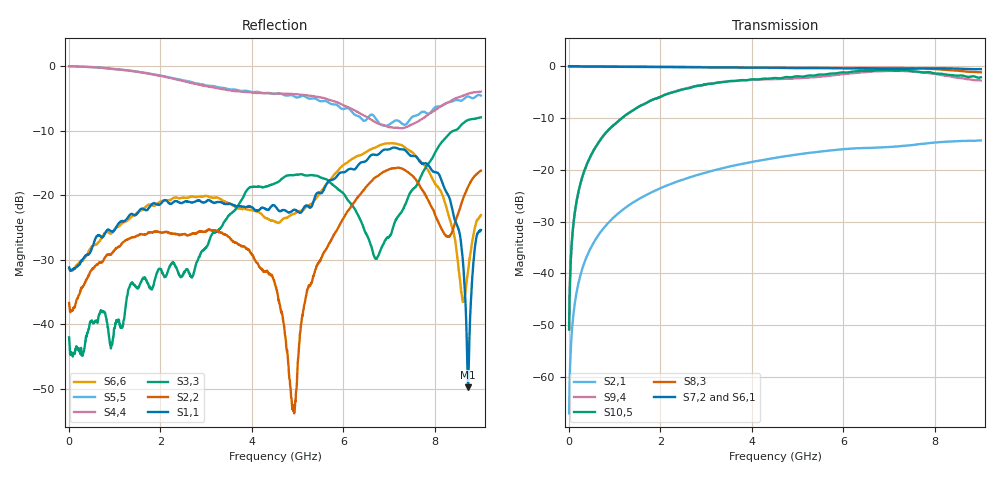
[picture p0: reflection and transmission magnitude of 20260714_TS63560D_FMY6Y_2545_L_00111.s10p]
# GHz S DB R 50
! CMT, SN0916, 25263762, 26.7.0
! Date: 15.07.2026 13:36:52
! Data: Format
! Freq S1.1:dB/Ang S1.2:dB/Ang S1.3:dB/Ang S1.4:dB/Ang S1.5:dB/Ang S1.6:dB/Ang S1.7:dB/Ang S1.8:dB/Ang S1.9:dB/Ang S1.10:dB/Ang
!  S2.1:dB/Ang S2.2:dB/Ang S2.3:dB/Ang S2.4:dB/Ang S2.5:dB/Ang S2.6:dB/Ang S2.7:dB/Ang S2.8:dB/Ang S2.9:dB/Ang S2.10:dB/Ang
!  S3.1:dB/Ang S3.2:dB/Ang S3.3:dB/Ang S3.4:dB/Ang S3.5:dB/Ang S3.6:dB/Ang S3.7:dB/Ang S3.8:dB/Ang S3.9:dB/Ang S3.10:dB/Ang
!  S4.1:dB/Ang S4.2:dB/Ang S4.3:dB/Ang S4.4:dB/Ang S4.5:dB/Ang S4.6:dB/Ang S4.7:dB/Ang S4.8:dB/Ang S4.9:dB/Ang S4.10:dB/Ang
!  S5.1:dB/Ang S5.2:dB/Ang S5.3:dB/Ang S5.4:dB/Ang S5.5:dB/Ang S5.6:dB/Ang S5.7:dB/Ang S5.8:dB/Ang S5.9:dB/Ang S5.10:dB/Ang
!  S6.1:dB/Ang S6.2:dB/Ang S6.3:dB/Ang S6.4:dB/Ang S6.5:dB/Ang S6.6:dB/Ang S6.7:dB/Ang S6.8:dB/Ang S6.9:dB/Ang S6.10:dB/Ang
!  S7.1:dB/Ang S7.2:dB/Ang S7.3:dB/Ang S7.4:dB/Ang S7.5:dB/Ang S7.6:dB/Ang S7.7:dB/Ang S7.8:dB/Ang S7.9:dB/Ang S7.10:dB/Ang
!  S8.1:dB/Ang S8.2:dB/Ang S8.3:dB/Ang S8.4:dB/Ang S8.5:dB/Ang S8.6:dB/Ang S8.7:dB/Ang S8.8:dB/Ang S8.9:dB/Ang S8.10:dB/Ang
!  S9.1:dB/Ang S9.2:dB/Ang S9.3:dB/Ang S9.4:dB/Ang S9.5:dB/Ang S9.6:dB/Ang S9.7:dB/Ang S9.8:dB/Ang S9.9:dB/Ang S9.10:dB/Ang
!  S10.1:dB/Ang S10.2:dB/Ang S10.3:dB/Ang S10.4:dB/Ang S10.5:dB/Ang S10.6:dB/Ang S10.7:dB/Ang S10.8:dB/Ang S10.9:dB/Ang S10.10:dB/Ang
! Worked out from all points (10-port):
!   2001 points, 10 MHz to 9 GHz, reference 50 ohm
!   strongest paths, dB at 10 MHz, 2.257 GHz, 4.505 GHz, 6.753 GHz, 9 GHz:
!     S7,2: -0.1, -0.3, -0.4, -0.6, -0.6
!     S8,3: -0.1, -0.2, -0.4, -0.4, -1.3
!     S6,1: -0.2, -0.4, -0.5, -0.7, -0.6
!     S10,5: -50.8, -5.1, -2.4, -0.8, -2.2
!     S9,4: -50.8, -5.1, -2.6, -1.0, -2.8
!     S2,1: -66.9, -22.7, -17.7, -15.7, -14.4
!   lowest |S11| = -49.7 dB at 8.721 GHz (marker M1), VSWR 1.01, Z = 49.9 + j0.295 ohm
!   |S11| at or under -10 dB: start of sweep to end of sweep
